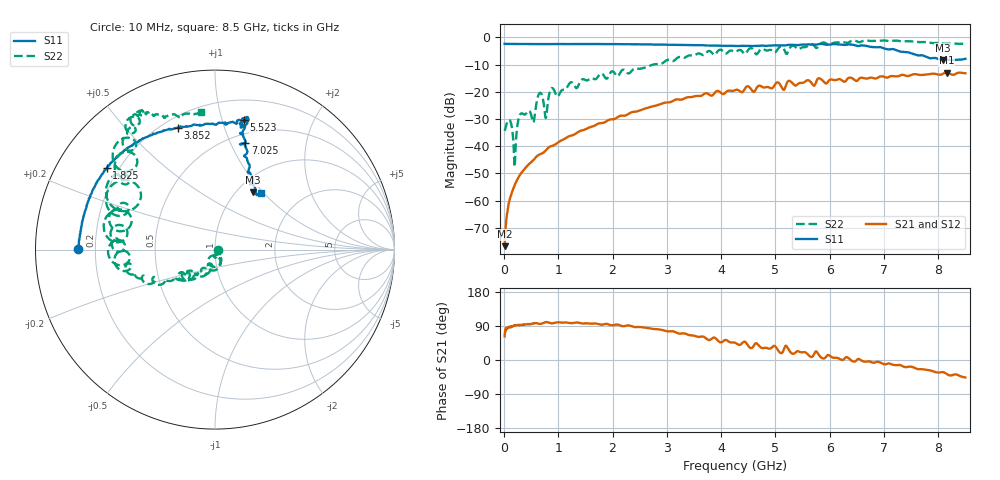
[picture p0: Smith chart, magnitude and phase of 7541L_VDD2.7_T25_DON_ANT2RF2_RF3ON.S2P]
!Agilent Technologies,E5071C,MY46417908,A.11.23
!Date: Wed Dec 09 17:17:59 2020
!Data & Calibration Information:
!Freq	S11:SOLT2(ON)	S21:SOLT2(ON)	S12:SOLT2(ON)	S22:SOLT2(ON)
!PortZ  Port1:50+j0  Port2:50+j0
!Above PortZ is port z conversion or system Z0 setting when saving the data.
!When reading, reference impedance value at option line is always used.
# Hz S dB R 50
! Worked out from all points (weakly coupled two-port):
!   1601 points, 10 MHz to 8.5 GHz, reference 50 ohm
!   highest |S21| = -12.90 dB at 8.155 GHz (marker M1); lowest = -76.7 dB at 10 MHz (marker M2)
!   lowest |S11| = -8.4 dB at 8.081 GHz (marker M3), VSWR 2.24, Z = 59 + j44 ohm
!   |S11| at or under -10 dB: nowhere
!   |S22| runs from -47.6 to -1.1 dB; largest |S21 - S12| = 0.0022
!   S11 on the Smith chart (normalised r, x): 10 MHz: 0.13, +0.00; 1.825 GHz: 0.15, +0.33; 3.852 GHz: 0.26, +0.71; 5.523 GHz: 0.37, +1.18; 7.025 GHz: 0.59, +1.14; 8.5 GHz: 1.27, +0.96
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1e7  -2.33 179.6  -76.73 62.2  -79.75 74.0  -34.31 0.1
6.30625e7  -2.38 178.5  -64.05 84.1  -64.01 84.8  -30.90 -24.8
1.055125e8  -2.39 177.5  -59.33 87.4  -59.46 87.9  -30.43 -58.7
1.957188e8  -2.41 175.5  -54.26 90.5  -54.40 92.0  -47.60 -52.3
3.018438e8  -2.44 173.1  -50.26 92.5  -50.29 92.7  -28.13 -52.3
5.353188e8  -2.43 168.1  -45.21 95.7  -45.17 95.9  -31.21 -82.5
6.573625e8  -2.43 165.5  -43.00 95.4  -42.99 95.2  -20.39 -88.6
7.687938e8  -2.44 163.3  -41.54 99.9  -41.50 99.9  -29.64 -94.4
8.749188e8  -2.43 161.0  -39.93 96.9  -39.90 96.9  -18.68 -92.4
9.916562e8  -2.43 158.4  -38.66 99.5  -38.68 99.4  -21.69 -105.2
1.426769e9  -2.42 150.2  -34.21 96.7  -34.21 96.7  -15.57 -115.6
1.824738e9  -2.43 142.9  -31.43 93.7  -31.43 93.7  -13.65 -139.7
2.843538e9  -2.60 126.5  -24.79 80.9  -24.80 80.9  -9.78 -149.3
3.851725e9  -2.97 106.9  -21.06 58.8  -21.06 58.7  -6.16 -178.6
4.255e9  -3.10 96.8  -19.36 45.6  -19.37 45.6  -5.29 174.1
5.523194e9  -2.62 77.5  -16.55 20.6  -16.53 20.6  -3.59 142.1
5.671769e9  -2.67 76.3  -16.96 8.2  -16.90 8.1  -2.50 135.0
7.024862e9  -4.17 74.1  -14.63 -11.5  -14.64 -11.4  -1.14 118.1
7.088538e9  -4.40 76.7  -14.54 -9.1  -14.58 -9.2  -1.37 117.8
8.080806e9  -8.35 56.5  -13.43 -31.7  -13.44 -31.7  -2.18 106.0
8.155094e9  -8.13 55.1  -12.90 -37.0  -12.93 -37.0  -2.33 104.8
8.5e9  -7.85 51.3  -13.18 -46.1  -13.26 -46.1  -2.28 95.9
